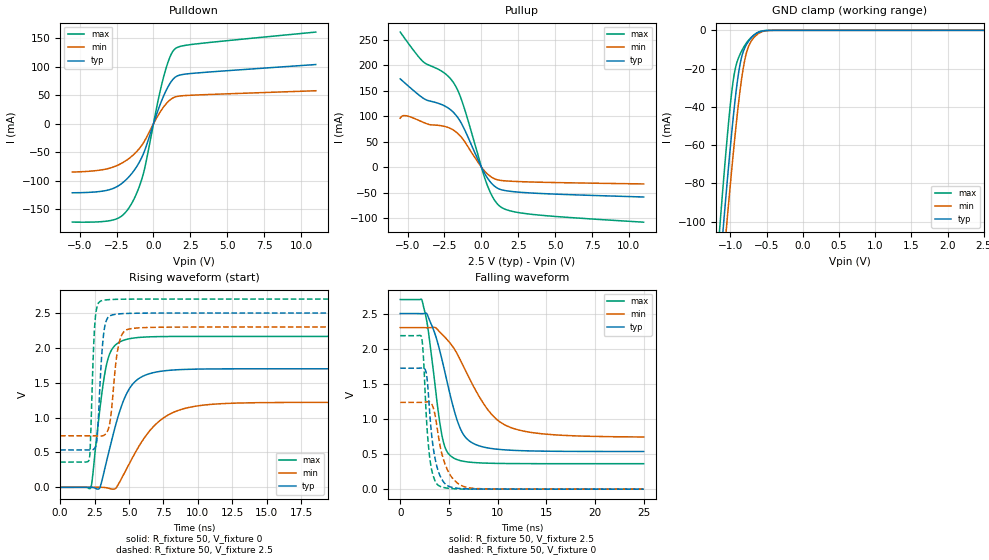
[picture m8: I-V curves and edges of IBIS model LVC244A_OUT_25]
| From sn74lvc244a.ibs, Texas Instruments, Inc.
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[Model]   LVC244A_OUT_25
Model_type  3-state
Enable   Active-Low
Vref =   0
Rref =   500
Cref =   30p
Vmeas =   1.25
| variable   typ   min   max
C_comp   3.84pF   3.46pF   4.32pF
| C_pullup   7.98pF   4.06pF   11.86pF
| C_pulldown   7.28pF   3.69pF   13.52pF
| C_tri-state   3.84pF   3.46pF   4.32pF
[Temperature Range]   40   100   -40
| Ambient temperature   25   85   -40
[Voltage range]   2.5   2.3   2.7
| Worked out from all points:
|   slope of the pulldown table from 0 to 0.375 V, typ, clamps not added: 13.2 ohm
|   slope of the pullup table from 0 to 0.375 V, typ, clamps not added: 18.9 ohm
|   GND clamp passes 1 mA (typ) near -0.61 V on its own axis
|   rising waveform, R_fixture 50, V_fixture 0: 20-80 % time 1.54ns typ, 2.6ns min, 838ps max; typ from 0 V to 1.7 V
|   falling waveform, R_fixture 50, V_fixture 2.5: 20-80 % time 2.18ns typ, 3.87ns min, 1.3ns max; typ from 2.5 V to 0.536 V
|   rising waveform, R_fixture 50, V_fixture 2.5: 20-80 % time 350ps typ, 497ps min, 252ps max; typ from 0.536 V to 2.5 V
|   falling waveform, R_fixture 50, V_fixture 0: 20-80 % time 846ps typ, 1.29ns min, 607ps max; typ from 1.72 V to 0 V
[GND Clamp]
| LVC244A_OUT_25
|   Voltage   I(typ)   I(min)   I(max)
-5.5V     -2.404A    -2.35A     -2.478A
-1.15V    -126.2mA   -144.8mA   -104.1mA
-1.09V    -98.87mA   -118.1mA   -75.86mA
-1.06V    -85.62mA   -105.1mA   -62.44mA
-1.045V   -79.13mA   -98.68mA   -55.99mA
-960mV    -44.92mA   -63.9mA    -25.79mA
-920mV    -31.3mA    -48.92mA   -17.97mA
-865mV    -17.32mA   -30.75mA   -12.31mA
-810mV    -9.84mA    -17mA      -8.374mA
-765mV    -6.571mA   -9.993mA   -5.882mA
-625mV    -1.251mA   -2.008mA   -1.13mA
2.5V      74.72pA    76.12nA    31.37pA
[Pulldown]
| LVC244A_OUT_25
|   Voltage   I(typ)   I(min)   I(max)
-5.5V     -120.8mA   -84.53mA   -172.2mA
-2.655V   -112.4mA   -75.06mA   -167.9mA
-2.055V   -102.6mA   -67.62mA   -159.4mA
-1.53V    -88.95mA   -58.14mA   -141.9mA
-1.055V   -71.56mA   -46.3mA    -116.4mA
-665mV    -51.45mA   -32.76mA   -85.52mA
310mV     23.77mA    14.55mA    40.43mA
785mV     54.37mA    32.73mA    91.27mA
1.15V     71.94mA    42.44mA    119mA
1.48V     81.76mA    47.14mA    131.7mA
2.83V     88.84mA    50.4mA     139.8mA
11V       103.8mA    57.91mA    160.7mA
[Pullup]
| LVC244A_OUT_25
|   Voltage   I(typ)   I(min)   I(max)
-5.5V     172.9mA    95.88mA    264.6mA
-5.1V     162.6mA    100.6mA    248.4mA
-3.985V   135.9mA    88.29mA    207.6mA
-2.495V   119.9mA    79.74mA    184.1mA
-1.76V    103mA      69.84mA    159.4mA
-1.145V   73.77mA    50.38mA    114.2mA
360mV     -19.12mA   -12.06mA   -32.41mA
805mV     -35.2mA    -21.67mA   -60.74mA
1.26V     -43.52mA   -25.91mA   -76.93mA
1.985V    -47.56mA   -27.67mA   -86.02mA
3.38V     -50.77mA   -29.2mA    -92.47mA
11V       -58.61mA   -33mA      -108mA
[Ramp]
| LVC244A_OUT_25
| variable   typ   min   max
dV/dt_r   1.04/1.55E-09   0.75/2.61E-09   1.31/8.44E-10
dV/dt_f   1.18/2.19E-09   0.94/3.88E-09   1.41/1.30E-09
R_load = 50
[Rising Waveform]
| LVC244A_OUT_25
R_fixture =   50
C_fixture =   0
L_fixture =   0
V_fixture =   0
V_fixture_min = 0
V_fixture_max = 0
|   Time   V(typ)   V(min)   V(max)
0s        336.2pV    3.631nV    125.9pV
2.22ns    1.218mV    117.1uV    -9.374mV
2.85ns    -17.54mV   1.276mV    1.063V
3.34ns    349.7mV    -5.319mV   1.734V
3.755ns   684.6mV    -24.55mV   1.978V
4.46ns    1.17V      127.8mV    2.098V
5.85ns    1.577V     630.8mV    2.151V
7.265ns   1.663V     960.4mV    2.162V
9.01ns    1.69V      1.13V      2.164V
24.99ns   1.7V       1.219V     2.164V
[Falling Waveform]
| LVC244A_OUT_25
R_fixture =   50
C_fixture =   0
L_fixture =   0
V_fixture =   2.5
V_fixture_min = 2.3
V_fixture_max = 2.7
|   Time   V(typ)   V(min)   V(max)
0s        2.5V       2.3V       2.7V
2.235ns   2.498V     2.3V       2.69V
2.84ns    2.465V     2.298V     2.294V
4.27ns    1.853V     2.207V     774.7mV
5.34ns    1.223V     2.039V     455.8mV
6.15ns    868.7mV    1.845V     407.5mV
6.98ns    699.5mV    1.61V      386.8mV
9.045ns   585.8mV    1.123V     369.7mV
10.91ns   558.1mV    903.1mV    365.3mV
24.99ns   536.1mV    742.6mV    362.5mV
[Rising Waveform]
| LVC244A_OUT_25
R_fixture =   50
C_fixture =   0
L_fixture =   0
V_fixture =   2.5
V_fixture_min = 2.3
V_fixture_max = 2.7
|   Time   V(typ)   V(min)   V(max)
0s        535.9mV    739mV      362.5mV
2.095ns   535.9mV    739.1mV    393.5mV
2.185ns   535.5mV    739.1mV    582.2mV
2.52ns    564.4mV    738.7mV    2.35V
2.705ns   766.8mV    737.7mV    2.609V
2.96ns    1.717V     736.2mV    2.672V
3.395ns   2.412V     789.2mV    2.689V
4.205ns   2.486V     2.001V     2.697V
4.825ns   2.494V     2.26V      2.699V
24.99ns   2.5V       2.3V       2.7V
[Falling Waveform]
| LVC244A_OUT_25
R_fixture =   50
C_fixture =   0
L_fixture =   0
V_fixture =   0
V_fixture_min = 0
V_fixture_max = 0
|   Time   V(typ)   V(min)   V(max)
0s        1.722V     1.235V     2.185V
2.185ns   1.725V     1.235V     2.165V
2.375ns   1.728V     1.236V     1.892V
2.675ns   1.65V      1.241V     1.046V
3.01ns    1.119V     1.243V     470.3mV
3.395ns   584.4mV    1.156V     187.2mV
3.965ns   231.3mV    715.8mV    49.67mV
5.03ns    38.36mV    225.5mV    11.09mV
6.775ns   4.932mV    27.39mV    1.441mV
24.99ns   47.49uV    121.1uV    19.4uV
